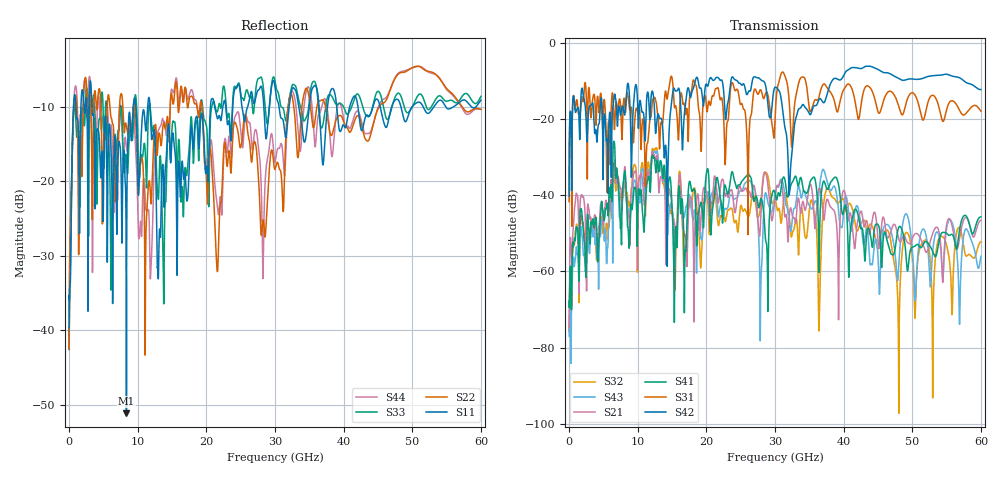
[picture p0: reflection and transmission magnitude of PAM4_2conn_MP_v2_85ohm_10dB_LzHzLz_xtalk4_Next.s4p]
! Info: Touchstone file created by Circ.  Input file=FAB50GbE_2conn_Midplane_Examax_Topo2_v2_85ohm_10dB_LzHzLz.circ
# Hz S RI R 50
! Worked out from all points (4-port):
!   6000 points, 10 MHz to 60 GHz, reference 50 ohm
!   strongest paths, dB at 10 MHz, 15.01 GHz, 30.01 GHz, 45.01 GHz, 60 GHz:
!     S42: -40.3, -14.5, -11.7, -7.0, -12.3
!     S31: -41.7, -9.3, -20.0, -18.1, -18.0
!     S41: -67.8, -43.3, -39.3, -47.7, -45.7
!     S21: -74.8, -43.4, -40.8, -51.7, -46.6
!     S43: -70.7, -43.8, -40.0, -56.1, -56.0
!     S32: -74.2, -44.3, -41.5, -54.0, -52.2
!   lowest |S11| = -51.2 dB at 8.36 GHz (marker M1), VSWR 1.01, Z = 50.1 + j0.234 ohm
!   |S11| at or under -10 dB: 3.336 GHz to 9.358 GHz (6.022 GHz wide, 94.9 % of centre); 11.8 GHz to 20.6 GHz (8.791 GHz wide, 54.3 % of centre); 42.09 GHz to 44.28 GHz (2.186 GHz wide, 5.06 % of centre)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
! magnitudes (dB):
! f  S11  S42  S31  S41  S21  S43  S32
! 10 MHz  -39.7  -40.3  -41.7  -67.8  -74.8  -70.7  -74.2
! 900 MHz  -8.7  -18.1  -17.7  -51.9  -42.1  -57.0  -49.6
! 8.36 GHz  -51.2  -13.6  -14.4  -40.3  -40.2  -42.0  -39.6
! 27.56 GHz  -7.7  -9.2  -13.5  -42.8  -48.1  -48.3  -45.8
! 32.17 GHz  -9.2  -36.6  -18.1  -38.5  -44.0  -48.6  -47.2
! 41.1 GHz  -9.4  -6.6  -11.6  -47.8  -45.6  -49.5  -42.7
! 60 GHz  -9.1  -12.3  -18.0  -45.7  -46.6  -56.0  -52.2
